| IBIS file stm32u535_545_lqfp64.ibs
[IBIS ver] 4.2
[File name] stm32u535_545_lqfp64.ibs
[File Rev] rev1.0
[Date]  11-09-2023
[Source] Data Created at STMicroelectronics
[Notes]  File originated from ELDO simulations.
[Disclaimer]  This information is for modeling purpose only and is
   not guaranteed. The information is subject to change without
   notice.
[Copyright] Copyright 2023 STMicroelectronics Inc.
|   Component stm32u535_545_lqfp64
[Component] stm32u535_545_lqfp64
[Manufacturer] STMicroelectronics
[Package]
| variable   typ   min   max
R_pkg  0  NA  NA
L_pkg  0  NA  NA
C_pkg  0  NA  NA
[Pin]   signal_name   model_name
1  VBAT  power
2  PC13  io8_100m_ft_v33
3  PC14-OSC32_IN  io8_100m_tamp_ft
4  PC15-OSC32_OUT  io8_100m_tamp_ft
5  PH0-OSC_IN  io8_100m_ft
6  PH1-OSC_OUT  io8_100m_ft
7  NRST  nc
8  PC0  io8_100m_hslv_i2c_ft
9  PC1  io8_166m_hslv_i2c_ft
10  PC2  io8_100m_hslv_ft
11  PC3  io8_100m_hslv_ft
12  VSSA  nc
13  VDDA  power
14  PA0  io8_100m_hslv_tamp_ft
15  PA1  io8_100m_hslv_tamp_ft
16  PA2  io8_100m_hslv_ft
17  PA3  io8_166m_hslv_ft
18  VSS  gnd
19  VDD  power
20  PA4  io8_100m_hslv_ft
21  PA5  io8_100m_ft
22  PA6  io8_100m_hslv_ft
23  PA7  io8_100m_hslv_i2c_ft
24  PC4  io8_100m_hslv_ft
25  PC5  io8_100m_tamp_ft
26  PB0  io8_100m_hslv_ft
27  PB1  io8_100m_hslv_ft
28  PB2  io8_100m_hslv_tamp_ft
29  PB10  io8_166m_hslv_i2c_ft
30  VCAP  nc
31  VSS  gnd
32  VDD  power
33  PB12  io8_166m_hslv_ft
34  PB13  io8_100m_i2c_ft
35  PB14  io8_100m_i2c_ft
36  PB15  io8_100m_ft
37  PC6  io8_100m_hslv_ft
38  PC7  io8_100m_hslv_ft
39  PC8  io8_100m_hslv_ft
40  PC9  io8_100m_hslv_ft
41  PA8  io8_166m_hslv_ft
42  PA9  io8_100m_ft
43  PA10  io8_100m_ft
44  PA11  io8_usb_ft
45  PA12  io8_usb_ft
46  PA13  io8_100m_ft
47  VSS  gnd
48  VDDUSB  power
49  PA14  io8_100m_ft
50  PA15  io8_100m_ft
51  PC10  io8_100m_hslv_ft
52  PC11  io8_100m_hslv_ft
53  PC12  io8_166m_hslv_ft
54  PD2  io8_100m_hslv_ft
55  PB3  io8_100m_i2c_ft
56  PB4  io8_100m_i2c_ft
57  PB5  io8_166m_hslv_ft
58  PB6  io8_100m_i2c_ft
59  PB7  io8_166m_hslv_i2c_ft
60  PH3-BOOT0  io8_100m_ft
61  PB8  io8_100m_hslv_i2c_ft
62  PB9  io8_100m_hslv_i2c_ft
63  VSS  gnd
64  VDD  power
[Package Model]   455-lqfp-10x10-64-ldo-230425
[Pin Mapping]   pulldown_ref   pullup_ref   | Comment
1  nc  vsw
2  gndio  vddiom  | Depending on IO usage
| 2  gndio  vsw  | Depending on IO usage
3  gndio  vddiom  | Depending on IO usage
| 3  gndio  vsw  | Depending on IO usage
4  gndio  vddiom  | Depending on IO usage
| 4  gndio  vsw  | Depending on IO usage
5  gndio  vddiom
6  gndio  vddiom
7  nc nc
8  gndio  vddiom
9  gndio  vddiom
10  gndio  vddiom
11  gndio  vddiom
12  nc  nc
13  nc  vddiom
14  gndio  vddiom
15  gndio  vddiom
16  gndio  vddiom
17  gndio  vddiom
18  gndio  nc
19  nc  vddiom
20  gndio  vddiom
21  gndio  vddiom
22  gndio  vddiom
23  gndio  vddiom
24  gndio  vddiom
25  gndio  vddiom
26  gndio  vddiom
27  gndio  vddiom
28  gndio  vddiom
29  gndio  vddiom
30  nc  nc
31  gndio  nc
32  nc  vddiom
33  gndio  vddiom
34  gndio  vddiom
35  gndio  vddiom
36  gndio  vddiom
37  gndio  vddiom
38  gndio  vddiom
39  gndio  vddiom
40  gndio  vddiom
41  gndio  vddiom
42  gndio  vddiom  | Depending on IO usage
| 42  gndio  vddusb  | Depending on IO usage
43  gndio  vddiom  | Depending on IO usage
| 43  gndio  vddusb  | Depending on IO usage
44  gndio  vddiom  | Depending on IO usage
| 44  gndio  vddusb  | Depending on IO usage
45  gndio  vddiom  | Depending on IO usage
| 45  gndio  vddusb  | Depending on IO usage
46  gndio  vddiom  | Depending on IO usage
| 46  gndio  vddusb  | Depending on IO usage
47  gndio  nc
48  nc  vddusb
49  gndio  vddiom
50  gndio  vddiom
51  gndio  vddiom
52  gndio  vddiom
53  gndio  vddiom
54  gndio  vddiom
55  gndio  vddiom
56  gndio  vddiom
57  gndio  vddiom
58  gndio  vddiom
59  gndio  vddiom
60  gndio  vddiom
61  gndio  vddiom
62  gndio  vddiom
63  gndio  nc
64  nc  vddiom
[Model Selector] io8_100m_ft
io8_100m_ft_hs_1v2  "IO8_FT 100MHz high speed @ 1.2V"
io8_100m_ft_fs_1v2  "IO8_FT 100MHz fast speed @ 1.2V"
io8_100m_ft_fs_pd_1v2  "IO8_FT 100MHz fast speed @ 1.2V pulldown"
io8_100m_ft_ms_1v2  "IO8_FT 100MHz med speed @ 1.2V"
io8_100m_ft_ms_pd_1v2  "IO8_FT 100MHz med speed @ 1.2V pulldown"
io8_100m_ft_ls_1v2  "IO8_FT 100MHz low speed @ 1.2V"
io8_100m_ft_ls_pd_1v2  "IO8_FT 100MHz low speed @ 1.2V pulldown"
io8_100m_ft_hs_1v8  "IO8_FT 100MHz high speed @ 1.8V"
io8_100m_ft_hs_pd_1v8  "IO8_FT 100MHz high speed @ 1.8V pulldown"
io8_100m_ft_fs_1v8  "IO8_FT 100MHz fast speed @ 1.8V"
io8_100m_ft_fs_pd_1v8  "IO8_FT 100MHz fast speed @ 1.8V pulldown"
io8_100m_ft_ms_1v8  "IO8_FT 100MHz med speed @ 1.8V"
io8_100m_ft_ms_pd_1v8  "IO8_FT 100MHz med speed @ 1.8V pulldown"
io8_100m_ft_ls_1v8  "IO8_FT 100MHz low speed @ 1.8V"
io8_100m_ft_ls_pd_1v8  "IO8_FT 100MHz low speed @ 1.8V pulldown"
io8_100m_ft_hs_3v3  "IO8_FT 100MHz high speed @ 3.3V"
io8_100m_ft_hs_pd_3v3  "IO8_FT 100MHz high speed @ 3.3V pulldown"
io8_100m_ft_fs_3v3  "IO8_FT 100MHz fast speed @ 3.3V"
io8_100m_ft_fs_pd_3v3  "IO8_FT 100MHz fast speed @ 3.3V pulldown"
io8_100m_ft_ms_3v3  "IO8_FT 100MHz med speed @ 3.3V"
io8_100m_ft_ms_pd_3v3  "IO8_FT 100MHz med speed @ 3.3V pulldown"
io8_100m_ft_ls_3v3  "IO8_FT 100MHz low speed @ 3.3V"
io8_100m_ft_ls_pd_3v3  "IO8_FT 100MHz low speed @ 3.3V pulldown"
[Model Selector] io8_100m_hslv_ft
io8_100m_ft_hs_1v2  "IO8_FT 100MHz high speed @ 1.2V"
io8_100m_ft_hs_pu_1v2  "IO8_FT 100MHz high speed @ 1.2V pullup"
io8_100m_ft_hs_pd_1v2  "IO8_FT 100MHz high speed @ 1.2V pulldown"
io8_100m_ft_fs_1v2  "IO8_FT 100MHz fast speed @ 1.2V"
io8_100m_ft_fs_pu_1v2  "IO8_FT 100MHz fast speed @ 1.2V pullup"
io8_100m_ft_fs_pd_1v2  "IO8_FT 100MHz fast speed @ 1.2V pulldown"
io8_100m_ft_ms_1v2  "IO8_FT 100MHz med speed @ 1.2V"
io8_100m_ft_ms_pu_1v2  "IO8_FT 100MHz med speed @ 1.2V pullup"
io8_100m_ft_ms_pd_1v2  "IO8_FT 100MHz med speed @ 1.2V pulldown"
io8_100m_ft_ls_1v2  "IO8_FT 100MHz low speed @ 1.2V"
io8_100m_ft_ls_pu_1v2  "IO8_FT 100MHz low speed @ 1.2V pullup"
io8_100m_ft_ls_pd_1v2  "IO8_FT 100MHz low speed @ 1.2V pulldown"
io8_100m_ft_hs_1v8  "IO8_FT 100MHz high speed @ 1.8V"
io8_100m_ft_hs_pu_1v8  "IO8_FT 100MHz high speed @ 1.8V pullup"
io8_100m_ft_hs_pd_1v8  "IO8_FT 100MHz high speed @ 1.8V pulldown"
io8_100m_ft_fs_1v8  "IO8_FT 100MHz fast speed @ 1.8V"
io8_100m_ft_fs_pu_1v8  "IO8_FT 100MHz fast speed @ 1.8V pullup"
io8_100m_ft_fs_pd_1v8  "IO8_FT 100MHz fast speed @ 1.8V pulldown"
io8_100m_ft_ms_1v8  "IO8_FT 100MHz med speed @ 1.8V"
io8_100m_ft_ms_pu_1v8  "IO8_FT 100MHz med speed @ 1.8V pullup"
io8_100m_ft_ms_pd_1v8  "IO8_FT 100MHz med speed @ 1.8V pulldown"
io8_100m_ft_ls_1v8  "IO8_FT 100MHz low speed @ 1.8V"
io8_100m_ft_ls_pu_1v8  "IO8_FT 100MHz low speed @ 1.8V pullup"
io8_100m_ft_ls_pd_1v8  "IO8_FT 100MHz low speed @ 1.8V pulldown"
io8_100m_ft_hs_3v3  "IO8_FT 100MHz high speed @ 3.3V"
io8_100m_ft_hs_pu_3v3  "IO8_FT 100MHz high speed @ 3.3V pullup"
io8_100m_ft_hs_pd_3v3  "IO8_FT 100MHz high speed @ 3.3V pulldown"
io8_100m_ft_fs_3v3  "IO8_FT 100MHz fast speed @ 3.3V"
io8_100m_ft_fs_pu_3v3  "IO8_FT 100MHz fast speed @ 3.3V pullup"
io8_100m_ft_fs_pd_3v3  "IO8_FT 100MHz fast speed @ 3.3V pulldown"
io8_100m_ft_ms_3v3  "IO8_FT 100MHz med speed @ 3.3V"
io8_100m_ft_ms_pu_3v3  "IO8_FT 100MHz med speed @ 3.3V pullup"
io8_100m_ft_ms_pd_3v3  "IO8_FT 100MHz med speed @ 3.3V pulldown"
io8_100m_ft_ls_3v3  "IO8_FT 100MHz low speed @ 3.3V"
io8_100m_ft_ls_pu_3v3  "IO8_FT 100MHz low speed @ 3.3V pullup"
io8_100m_ft_ls_pd_3v3  "IO8_FT 100MHz low speed @ 3.3V pulldown"
io8_100m_hslv_ft_hs_1v2  "IO8_FT 100MHz HSLV high speed @ 1.2V"
io8_100m_hslv_ft_hs_pu_1v2  "IO8_FT 100MHz HSLV high speed @ 1.2V pullup"
io8_100m_hslv_ft_hs_pd_1v2  "IO8_FT 100MHz HSLV high speed @ 1.2V pulldown"
io8_100m_hslv_ft_fs_1v2  "IO8_FT 100MHz HSLV fast speed @ 1.2V"
io8_100m_hslv_ft_fs_pu_1v2  "IO8_FT 100MHz HSLV fast speed @ 1.2V pullup"
io8_100m_hslv_ft_fs_pd_1v2  "IO8_FT 100MHz HSLV fast speed @ 1.2V pulldown"
io8_100m_hslv_ft_ms_1v2  "IO8_FT 100MHz HSLV med speed @ 1.2V"
io8_100m_hslv_ft_ms_pu_1v2  "IO8_FT 100MHz HSLV med speed @ 1.2V pullup"
io8_100m_hslv_ft_ms_pd_1v2  "IO8_FT 100MHz HSLV med speed @ 1.2V pulldown"
io8_100m_hslv_ft_ls_1v2  "IO8_FT 100MHz HSLV low speed @ 1.2V"
io8_100m_hslv_ft_ls_pu_1v2  "IO8_FT 100MHz HSLV low speed @ 1.2V pullup"
io8_100m_hslv_ft_ls_pd_1v2  "IO8_FT 100MHz HSLV low speed @ 1.2V pulldown"
io8_100m_hslv_ft_hs_1v8  "IO8_FT 100MHz HSLV high speed @ 1.8V"
io8_100m_hslv_ft_hs_pu_1v8  "IO8_FT 100MHz HSLV high speed @ 1.8V pullup"
io8_100m_hslv_ft_hs_pd_1v8  "IO8_FT 100MHz HSLV high speed @ 1.8V pulldown"
io8_100m_hslv_ft_fs_1v8  "IO8_FT 100MHz HSLV fast speed @ 1.8V"
io8_100m_hslv_ft_fs_pu_1v8  "IO8_FT 100MHz HSLV fast speed @ 1.8V pullup"
io8_100m_hslv_ft_fs_pd_1v8  "IO8_FT 100MHz HSLV fast speed @ 1.8V pulldown"
io8_100m_hslv_ft_ms_1v8  "IO8_FT 100MHz HSLV med speed @ 1.8V"
io8_100m_hslv_ft_ms_pu_1v8  "IO8_FT 100MHz HSLV med speed @ 1.8V pullup"
io8_100m_hslv_ft_ms_pd_1v8  "IO8_FT 100MHz HSLV med speed @ 1.8V pulldown"
io8_100m_hslv_ft_ls_1v8  "IO8_FT 100MHz HSLV low speed @ 1.8V"
io8_100m_hslv_ft_ls_pu_1v8  "IO8_FT 100MHz HSLV low speed @ 1.8V pullup"
io8_100m_hslv_ft_ls_pd_1v8  "IO8_FT 100MHz HSLV low speed @ 1.8V pulldown"
io8_100m_hslv_ft_hs_2v5  "IO8_FT 100MHz HSLV high speed @ 2.5V"
io8_100m_hslv_ft_hs_pu_2v5  "IO8_FT 100MHz HSLV high speed @ 2.5V pullup"
io8_100m_hslv_ft_hs_pd_2v5  "IO8_FT 100MHz HSLV high speed @ 2.5V pulldown"
io8_100m_hslv_ft_fs_2v5  "IO8_FT 100MHz HSLV fast speed @ 2.5V"
io8_100m_hslv_ft_fs_pu_2v5  "IO8_FT 100MHz HSLV fast speed @ 2.5V pullup"
io8_100m_hslv_ft_fs_pd_2v5  "IO8_FT 100MHz HSLV fast speed @ 2.5V pulldown"
io8_100m_hslv_ft_ms_2v5  "IO8_FT 100MHz HSLV med speed @ 2.5V"
io8_100m_hslv_ft_ms_pu_2v5  "IO8_FT 100MHz HSLV med speed @ 2.5V pullup"
io8_100m_hslv_ft_ms_pd_2v5  "IO8_FT 100MHz HSLV med speed @ 2.5V pulldown"
io8_100m_hslv_ft_ls_2v5  "IO8_FT 100MHz HSLV low speed @ 2.5V"
io8_100m_hslv_ft_ls_pu_2v5  "IO8_FT 100MHz HSLV low speed @ 2.5V pullup"
io8_100m_hslv_ft_ls_pd_2v5  "IO8_FT 100MHz HSLV low speed @ 2.5V pulldown"
[Model Selector] io8_100m_hslv_i2c_ft
io8_100m_ft_hs_1v2  "IO8_FT 100MHz high speed @ 1.2V"
io8_100m_ft_hs_pu_1v2  "IO8_FT 100MHz high speed @ 1.2V pullup"
io8_100m_ft_hs_pd_1v2  "IO8_FT 100MHz high speed @ 1.2V pulldown"
io8_100m_ft_fs_1v2  "IO8_FT 100MHz fast speed @ 1.2V"
io8_100m_ft_fs_pu_1v2  "IO8_FT 100MHz fast speed @ 1.2V pullup"
io8_100m_ft_fs_pd_1v2  "IO8_FT 100MHz fast speed @ 1.2V pulldown"
io8_100m_ft_ms_1v2  "IO8_FT 100MHz med speed @ 1.2V"
io8_100m_ft_ms_pu_1v2  "IO8_FT 100MHz med speed @ 1.2V pullup"
io8_100m_ft_ms_pd_1v2  "IO8_FT 100MHz med speed @ 1.2V pulldown"
io8_100m_ft_ls_1v2  "IO8_FT 100MHz low speed @ 1.2V"
io8_100m_ft_ls_pu_1v2  "IO8_FT 100MHz low speed @ 1.2V pullup"
io8_100m_ft_ls_pd_1v2  "IO8_FT 100MHz low speed @ 1.2V pulldown"
io8_100m_ft_hs_1v8  "IO8_FT 100MHz high speed @ 1.8V"
io8_100m_ft_hs_pu_1v8  "IO8_FT 100MHz high speed @ 1.8V pullup"
io8_100m_ft_hs_pd_1v8  "IO8_FT 100MHz high speed @ 1.8V pulldown"
io8_100m_ft_fs_1v8  "IO8_FT 100MHz fast speed @ 1.8V"
io8_100m_ft_fs_pu_1v8  "IO8_FT 100MHz fast speed @ 1.8V pullup"
io8_100m_ft_fs_pd_1v8  "IO8_FT 100MHz fast speed @ 1.8V pulldown"
io8_100m_ft_ms_1v8  "IO8_FT 100MHz med speed @ 1.8V"
io8_100m_ft_ms_pu_1v8  "IO8_FT 100MHz med speed @ 1.8V pullup"
io8_100m_ft_ms_pd_1v8  "IO8_FT 100MHz med speed @ 1.8V pulldown"
io8_100m_ft_ls_1v8  "IO8_FT 100MHz low speed @ 1.8V"
io8_100m_ft_ls_pu_1v8  "IO8_FT 100MHz low speed @ 1.8V pullup"
io8_100m_ft_ls_pd_1v8  "IO8_FT 100MHz low speed @ 1.8V pulldown"
io8_100m_ft_hs_3v3  "IO8_FT 100MHz high speed @ 3.3V"
io8_100m_ft_hs_pu_3v3  "IO8_FT 100MHz high speed @ 3.3V pullup"
io8_100m_ft_hs_pd_3v3  "IO8_FT 100MHz high speed @ 3.3V pulldown"
io8_100m_ft_fs_3v3  "IO8_FT 100MHz fast speed @ 3.3V"
io8_100m_ft_fs_pu_3v3  "IO8_FT 100MHz fast speed @ 3.3V pullup"
io8_100m_ft_fs_pd_3v3  "IO8_FT 100MHz fast speed @ 3.3V pulldown"
io8_100m_ft_ms_3v3  "IO8_FT 100MHz med speed @ 3.3V"
io8_100m_ft_ms_pu_3v3  "IO8_FT 100MHz med speed @ 3.3V pullup"
io8_100m_ft_ms_pd_3v3  "IO8_FT 100MHz med speed @ 3.3V pulldown"
io8_100m_ft_ls_3v3  "IO8_FT 100MHz low speed @ 3.3V"
io8_100m_ft_ls_pu_3v3  "IO8_FT 100MHz low speed @ 3.3V pullup"
io8_100m_ft_ls_pd_3v3  "IO8_FT 100MHz low speed @ 3.3V pulldown"
io8_100m_hslv_ft_hs_1v2  "IO8_FT 100MHz HSLV high speed @ 1.2V"
io8_100m_hslv_ft_hs_pu_1v2  "IO8_FT 100MHz HSLV high speed @ 1.2V pullup"
io8_100m_hslv_ft_hs_pd_1v2  "IO8_FT 100MHz HSLV high speed @ 1.2V pulldown"
io8_100m_hslv_ft_fs_1v2  "IO8_FT 100MHz HSLV fast speed @ 1.2V"
io8_100m_hslv_ft_fs_pu_1v2  "IO8_FT 100MHz HSLV fast speed @ 1.2V pullup"
io8_100m_hslv_ft_fs_pd_1v2  "IO8_FT 100MHz HSLV fast speed @ 1.2V pulldown"
io8_100m_hslv_ft_ms_1v2  "IO8_FT 100MHz HSLV med speed @ 1.2V"
io8_100m_hslv_ft_ms_pu_1v2  "IO8_FT 100MHz HSLV med speed @ 1.2V pullup"
io8_100m_hslv_ft_ms_pd_1v2  "IO8_FT 100MHz HSLV med speed @ 1.2V pulldown"
io8_100m_hslv_ft_ls_1v2  "IO8_FT 100MHz HSLV low speed @ 1.2V"
io8_100m_hslv_ft_ls_pu_1v2  "IO8_FT 100MHz HSLV low speed @ 1.2V pullup"
io8_100m_hslv_ft_ls_pd_1v2  "IO8_FT 100MHz HSLV low speed @ 1.2V pulldown"
io8_100m_hslv_ft_hs_1v8  "IO8_FT 100MHz HSLV high speed @ 1.8V"
io8_100m_hslv_ft_hs_pu_1v8  "IO8_FT 100MHz HSLV high speed @ 1.8V pullup"
io8_100m_hslv_ft_hs_pd_1v8  "IO8_FT 100MHz HSLV high speed @ 1.8V pulldown"
io8_100m_hslv_ft_fs_1v8  "IO8_FT 100MHz HSLV fast speed @ 1.8V"
io8_100m_hslv_ft_fs_pu_1v8  "IO8_FT 100MHz HSLV fast speed @ 1.8V pullup"
io8_100m_hslv_ft_fs_pd_1v8  "IO8_FT 100MHz HSLV fast speed @ 1.8V pulldown"
io8_100m_hslv_ft_ms_1v8  "IO8_FT 100MHz HSLV med speed @ 1.8V"
io8_100m_hslv_ft_ms_pu_1v8  "IO8_FT 100MHz HSLV med speed @ 1.8V pullup"
io8_100m_hslv_ft_ms_pd_1v8  "IO8_FT 100MHz HSLV med speed @ 1.8V pulldown"
io8_100m_hslv_ft_ls_1v8  "IO8_FT 100MHz HSLV low speed @ 1.8V"
io8_100m_hslv_ft_ls_pu_1v8  "IO8_FT 100MHz HSLV low speed @ 1.8V pullup"
io8_100m_hslv_ft_ls_pd_1v8  "IO8_FT 100MHz HSLV low speed @ 1.8V pulldown"
io8_100m_hslv_ft_hs_2v5  "IO8_FT 100MHz HSLV high speed @ 2.5V"
io8_100m_hslv_ft_hs_pu_2v5  "IO8_FT 100MHz HSLV high speed @ 2.5V pullup"
io8_100m_hslv_ft_hs_pd_2v5  "IO8_FT 100MHz HSLV high speed @ 2.5V pulldown"
io8_100m_hslv_ft_fs_2v5  "IO8_FT 100MHz HSLV fast speed @ 2.5V"
io8_100m_hslv_ft_fs_pu_2v5  "IO8_FT 100MHz HSLV fast speed @ 2.5V pullup"
io8_100m_hslv_ft_fs_pd_2v5  "IO8_FT 100MHz HSLV fast speed @ 2.5V pulldown"
io8_100m_hslv_ft_ms_2v5  "IO8_FT 100MHz HSLV med speed @ 2.5V"
io8_100m_hslv_ft_ms_pu_2v5  "IO8_FT 100MHz HSLV med speed @ 2.5V pullup"
io8_100m_hslv_ft_ms_pd_2v5  "IO8_FT 100MHz HSLV med speed @ 2.5V pulldown"
io8_100m_hslv_ft_ls_2v5  "IO8_FT 100MHz HSLV low speed @ 2.5V"
io8_100m_hslv_ft_ls_pu_2v5  "IO8_FT 100MHz HSLV low speed @ 2.5V pullup"
io8_100m_hslv_ft_ls_pd_2v5  "IO8_FT 100MHz HSLV low speed @ 2.5V pulldown"
[Model Selector] io8_100m_hslv_tamp_ft
io8_100m_ft_hs_1v2  "IO8_FT 100MHz high speed @ 1.2V"
io8_100m_ft_hs_pu_1v2  "IO8_FT 100MHz high speed @ 1.2V pullup"
io8_100m_ft_hs_pd_1v2  "IO8_FT 100MHz high speed @ 1.2V pulldown"
io8_100m_ft_fs_1v2  "IO8_FT 100MHz fast speed @ 1.2V"
io8_100m_ft_fs_pu_1v2  "IO8_FT 100MHz fast speed @ 1.2V pullup"
io8_100m_ft_fs_pd_1v2  "IO8_FT 100MHz fast speed @ 1.2V pulldown"
io8_100m_ft_ms_1v2  "IO8_FT 100MHz med speed @ 1.2V"
io8_100m_ft_ms_pu_1v2  "IO8_FT 100MHz med speed @ 1.2V pullup"
io8_100m_ft_ms_pd_1v2  "IO8_FT 100MHz med speed @ 1.2V pulldown"
io8_100m_ft_ls_1v2  "IO8_FT 100MHz low speed @ 1.2V"
io8_100m_ft_ls_pu_1v2  "IO8_FT 100MHz low speed @ 1.2V pullup"
io8_100m_ft_ls_pd_1v2  "IO8_FT 100MHz low speed @ 1.2V pulldown"
io8_100m_ft_hs_1v8  "IO8_FT 100MHz high speed @ 1.8V"
io8_100m_ft_hs_pu_1v8  "IO8_FT 100MHz high speed @ 1.8V pullup"
io8_100m_ft_hs_pd_1v8  "IO8_FT 100MHz high speed @ 1.8V pulldown"
io8_100m_ft_fs_1v8  "IO8_FT 100MHz fast speed @ 1.8V"
io8_100m_ft_fs_pu_1v8  "IO8_FT 100MHz fast speed @ 1.8V pullup"
io8_100m_ft_fs_pd_1v8  "IO8_FT 100MHz fast speed @ 1.8V pulldown"
io8_100m_ft_ms_1v8  "IO8_FT 100MHz med speed @ 1.8V"
io8_100m_ft_ms_pu_1v8  "IO8_FT 100MHz med speed @ 1.8V pullup"
io8_100m_ft_ms_pd_1v8  "IO8_FT 100MHz med speed @ 1.8V pulldown"
io8_100m_ft_ls_1v8  "IO8_FT 100MHz low speed @ 1.8V"
io8_100m_ft_ls_pu_1v8  "IO8_FT 100MHz low speed @ 1.8V pullup"
io8_100m_ft_ls_pd_1v8  "IO8_FT 100MHz low speed @ 1.8V pulldown"
io8_100m_ft_hs_3v3  "IO8_FT 100MHz high speed @ 3.3V"
io8_100m_ft_hs_pu_3v3  "IO8_FT 100MHz high speed @ 3.3V pullup"
io8_100m_ft_hs_pd_3v3  "IO8_FT 100MHz high speed @ 3.3V pulldown"
io8_100m_ft_fs_3v3  "IO8_FT 100MHz fast speed @ 3.3V"
io8_100m_ft_fs_pu_3v3  "IO8_FT 100MHz fast speed @ 3.3V pullup"
io8_100m_ft_fs_pd_3v3  "IO8_FT 100MHz fast speed @ 3.3V pulldown"
io8_100m_ft_ms_3v3  "IO8_FT 100MHz med speed @ 3.3V"
io8_100m_ft_ms_pu_3v3  "IO8_FT 100MHz med speed @ 3.3V pullup"
io8_100m_ft_ms_pd_3v3  "IO8_FT 100MHz med speed @ 3.3V pulldown"
io8_100m_ft_ls_3v3  "IO8_FT 100MHz low speed @ 3.3V"
io8_100m_ft_ls_pu_3v3  "IO8_FT 100MHz low speed @ 3.3V pullup"
io8_100m_ft_ls_pd_3v3  "IO8_FT 100MHz low speed @ 3.3V pulldown"
io8_100m_hslv_ft_hs_1v2  "IO8_FT 100MHz HSLV high speed @ 1.2V"
io8_100m_hslv_ft_hs_pu_1v2  "IO8_FT 100MHz HSLV high speed @ 1.2V pullup"
io8_100m_hslv_ft_hs_pd_1v2  "IO8_FT 100MHz HSLV high speed @ 1.2V pulldown"
io8_100m_hslv_ft_fs_1v2  "IO8_FT 100MHz HSLV fast speed @ 1.2V"
io8_100m_hslv_ft_fs_pu_1v2  "IO8_FT 100MHz HSLV fast speed @ 1.2V pullup"
io8_100m_hslv_ft_fs_pd_1v2  "IO8_FT 100MHz HSLV fast speed @ 1.2V pulldown"
io8_100m_hslv_ft_ms_1v2  "IO8_FT 100MHz HSLV med speed @ 1.2V"
io8_100m_hslv_ft_ms_pu_1v2  "IO8_FT 100MHz HSLV med speed @ 1.2V pullup"
io8_100m_hslv_ft_ms_pd_1v2  "IO8_FT 100MHz HSLV med speed @ 1.2V pulldown"
io8_100m_hslv_ft_ls_1v2  "IO8_FT 100MHz HSLV low speed @ 1.2V"
io8_100m_hslv_ft_ls_pu_1v2  "IO8_FT 100MHz HSLV low speed @ 1.2V pullup"
io8_100m_hslv_ft_ls_pd_1v2  "IO8_FT 100MHz HSLV low speed @ 1.2V pulldown"
io8_100m_hslv_ft_hs_1v8  "IO8_FT 100MHz HSLV high speed @ 1.8V"
io8_100m_hslv_ft_hs_pu_1v8  "IO8_FT 100MHz HSLV high speed @ 1.8V pullup"
io8_100m_hslv_ft_hs_pd_1v8  "IO8_FT 100MHz HSLV high speed @ 1.8V pulldown"
io8_100m_hslv_ft_fs_1v8  "IO8_FT 100MHz HSLV fast speed @ 1.8V"
io8_100m_hslv_ft_fs_pu_1v8  "IO8_FT 100MHz HSLV fast speed @ 1.8V pullup"
io8_100m_hslv_ft_fs_pd_1v8  "IO8_FT 100MHz HSLV fast speed @ 1.8V pulldown"
io8_100m_hslv_ft_ms_1v8  "IO8_FT 100MHz HSLV med speed @ 1.8V"
io8_100m_hslv_ft_ms_pu_1v8  "IO8_FT 100MHz HSLV med speed @ 1.8V pullup"
io8_100m_hslv_ft_ms_pd_1v8  "IO8_FT 100MHz HSLV med speed @ 1.8V pulldown"
io8_100m_hslv_ft_ls_1v8  "IO8_FT 100MHz HSLV low speed @ 1.8V"
io8_100m_hslv_ft_ls_pu_1v8  "IO8_FT 100MHz HSLV low speed @ 1.8V pullup"
io8_100m_hslv_ft_ls_pd_1v8  "IO8_FT 100MHz HSLV low speed @ 1.8V pulldown"
io8_100m_hslv_ft_hs_2v5  "IO8_FT 100MHz HSLV high speed @ 2.5V"
io8_100m_hslv_ft_hs_pu_2v5  "IO8_FT 100MHz HSLV high speed @ 2.5V pullup"
io8_100m_hslv_ft_hs_pd_2v5  "IO8_FT 100MHz HSLV high speed @ 2.5V pulldown"
io8_100m_hslv_ft_fs_2v5  "IO8_FT 100MHz HSLV fast speed @ 2.5V"
io8_100m_hslv_ft_fs_pu_2v5  "IO8_FT 100MHz HSLV fast speed @ 2.5V pullup"
io8_100m_hslv_ft_fs_pd_2v5  "IO8_FT 100MHz HSLV fast speed @ 2.5V pulldown"
io8_100m_hslv_ft_ms_2v5  "IO8_FT 100MHz HSLV med speed @ 2.5V"
io8_100m_hslv_ft_ms_pu_2v5  "IO8_FT 100MHz HSLV med speed @ 2.5V pullup"
io8_100m_hslv_ft_ms_pd_2v5  "IO8_FT 100MHz HSLV med speed @ 2.5V pulldown"
io8_100m_hslv_ft_ls_2v5  "IO8_FT 100MHz HSLV low speed @ 2.5V"
io8_100m_hslv_ft_ls_pu_2v5  "IO8_FT 100MHz HSLV low speed @ 2.5V pullup"
io8_100m_hslv_ft_ls_pd_2v5  "IO8_FT 100MHz HSLV low speed @ 2.5V pulldown"
io8_ft_v33_hs_1v2  "IO8_FT_V33 high speed @ 1.2V"
io8_ft_v33_hs_pu_1v2  "IO8_FT_V33 high speed @ 1.2V pullup"
io8_ft_v33_hs_pd_1v2  "IO8_FT_V33 high speed @ 1.2V pulldown"
io8_ft_v33_fs_1v2  "IO8_FT_V33 fast speed @ 1.2V"
io8_ft_v33_fs_pu_1v2  "IO8_FT_V33 fast speed @ 1.2V pullup"
io8_ft_v33_fs_pd_1v2  "IO8_FT_V33 fast speed @ 1.2V pulldown"
io8_ft_v33_ms_1v2  "IO8_FT_V33 med speed @ 1.2V"
io8_ft_v33_ms_pu_1v2  "IO8_FT_V33 med speed @ 1.2V pullup"
io8_ft_v33_ms_pd_1v2  "IO8_FT_V33 med speed @ 1.2V pulldown"
io8_ft_v33_ls_1v2  "IO8_FT_V33 low speed @ 1.2V"
io8_ft_v33_ls_pu_1v2  "IO8_FT_V33 low speed @ 1.2V pullup"
io8_ft_v33_ls_pd_1v2  "IO8_FT_V33 low speed @ 1.2V pulldown"
io8_ft_v33_hs_1v8  "IO8_FT_V33 high speed @ 1.8V"
io8_ft_v33_hs_pu_1v8  "IO8_FT_V33 high speed @ 1.8V pullup"
io8_ft_v33_hs_pd_1v8  "IO8_FT_V33 high speed @ 1.8V pulldown"
io8_ft_v33_fs_1v8  "IO8_FT_V33 fast speed @ 1.8V"
io8_ft_v33_fs_pu_1v8  "IO8_FT_V33 fast speed @ 1.8V pullup"
io8_ft_v33_fs_pd_1v8  "IO8_FT_V33 fast speed @ 1.8V pulldown"
io8_ft_v33_ms_1v8  "IO8_FT_V33 med speed @ 1.8V"
io8_ft_v33_ms_pu_1v8  "IO8_FT_V33 med speed @ 1.8V pullup"
io8_ft_v33_ms_pd_1v8  "IO8_FT_V33 med speed @ 1.8V pulldown"
io8_ft_v33_ls_1v8  "IO8_FT_V33 low speed @ 1.8V"
io8_ft_v33_ls_pu_1v8  "IO8_FT_V33 low speed @ 1.8V pullup"
io8_ft_v33_ls_pd_1v8  "IO8_FT_V33 low speed @ 1.8V pulldown"
io8_ft_v33_hs_3v3  "IO8_FT_V33 high speed @ 3.3V"
io8_ft_v33_hs_pu_3v3  "IO8_FT_V33 high speed @ 3.3V pullup"
io8_ft_v33_hs_pd_3v3  "IO8_FT_V33 high speed @ 3.3V pulldown"
io8_ft_v33_fs_3v3  "IO8_FT_V33 fast speed @ 3.3V"
io8_ft_v33_fs_pu_3v3  "IO8_FT_V33 fast speed @ 3.3V pullup"
io8_ft_v33_fs_pd_3v3  "IO8_FT_V33 fast speed @ 3.3V pulldown"
io8_ft_v33_ms_3v3  "IO8_FT_V33 med speed @ 3.3V"
io8_ft_v33_ms_pu_3v3  "IO8_FT_V33 med speed @ 3.3V pullup"
io8_ft_v33_ms_pd_3v3  "IO8_FT_V33 med speed @ 3.3V pulldown"
io8_ft_v33_ls_3v3  "IO8_FT_V33 low speed @ 3.3V"
io8_ft_v33_ls_pu_3v3  "IO8_FT_V33 low speed @ 3.3V pullup"
io8_ft_v33_ls_pd_3v3  "IO8_FT_V33 low speed @ 3.3V pulldown"
[Model Selector] io8_100m_i2c_ft
io8_100m_ft_hs_1v2  "IO8_FT 100MHz high speed @ 1.2V"
io8_100m_ft_hs_pu_1v2  "IO8_FT 100MHz high speed @ 1.2V pullup"
io8_100m_ft_hs_pd_1v2  "IO8_FT 100MHz high speed @ 1.2V pulldown"
io8_100m_ft_fs_1v2  "IO8_FT 100MHz fast speed @ 1.2V"
io8_100m_ft_fs_pu_1v2  "IO8_FT 100MHz fast speed @ 1.2V pullup"
io8_100m_ft_fs_pd_1v2  "IO8_FT 100MHz fast speed @ 1.2V pulldown"
io8_100m_ft_ms_1v2  "IO8_FT 100MHz med speed @ 1.2V"
io8_100m_ft_ms_pu_1v2  "IO8_FT 100MHz med speed @ 1.2V pullup"
io8_100m_ft_ms_pd_1v2  "IO8_FT 100MHz med speed @ 1.2V pulldown"
io8_100m_ft_ls_1v2  "IO8_FT 100MHz low speed @ 1.2V"
io8_100m_ft_ls_pu_1v2  "IO8_FT 100MHz low speed @ 1.2V pullup"
io8_100m_ft_ls_pd_1v2  "IO8_FT 100MHz low speed @ 1.2V pulldown"
io8_100m_ft_hs_1v8  "IO8_FT 100MHz high speed @ 1.8V"
io8_100m_ft_hs_pu_1v8  "IO8_FT 100MHz high speed @ 1.8V pullup"
io8_100m_ft_hs_pd_1v8  "IO8_FT 100MHz high speed @ 1.8V pulldown"
io8_100m_ft_fs_1v8  "IO8_FT 100MHz fast speed @ 1.8V"
io8_100m_ft_fs_pu_1v8  "IO8_FT 100MHz fast speed @ 1.8V pullup"
io8_100m_ft_fs_pd_1v8  "IO8_FT 100MHz fast speed @ 1.8V pulldown"
io8_100m_ft_ms_1v8  "IO8_FT 100MHz med speed @ 1.8V"
io8_100m_ft_ms_pu_1v8  "IO8_FT 100MHz med speed @ 1.8V pullup"
io8_100m_ft_ms_pd_1v8  "IO8_FT 100MHz med speed @ 1.8V pulldown"
io8_100m_ft_ls_1v8  "IO8_FT 100MHz low speed @ 1.8V"
io8_100m_ft_ls_pu_1v8  "IO8_FT 100MHz low speed @ 1.8V pullup"
io8_100m_ft_ls_pd_1v8  "IO8_FT 100MHz low speed @ 1.8V pulldown"
io8_100m_ft_hs_3v3  "IO8_FT 100MHz high speed @ 3.3V"
io8_100m_ft_hs_pu_3v3  "IO8_FT 100MHz high speed @ 3.3V pullup"
io8_100m_ft_hs_pd_3v3  "IO8_FT 100MHz high speed @ 3.3V pulldown"
io8_100m_ft_fs_3v3  "IO8_FT 100MHz fast speed @ 3.3V"
io8_100m_ft_fs_pu_3v3  "IO8_FT 100MHz fast speed @ 3.3V pullup"
io8_100m_ft_fs_pd_3v3  "IO8_FT 100MHz fast speed @ 3.3V pulldown"
io8_100m_ft_ms_3v3  "IO8_FT 100MHz med speed @ 3.3V"
io8_100m_ft_ms_pu_3v3  "IO8_FT 100MHz med speed @ 3.3V pullup"
io8_100m_ft_ms_pd_3v3  "IO8_FT 100MHz med speed @ 3.3V pulldown"
io8_100m_ft_ls_3v3  "IO8_FT 100MHz low speed @ 3.3V"
io8_100m_ft_ls_pu_3v3  "IO8_FT 100MHz low speed @ 3.3V pullup"
io8_100m_ft_ls_pd_3v3  "IO8_FT 100MHz low speed @ 3.3V pulldown"
io8_100m_i2c_ft_1v2  "IO8_FT 100MHz I2C @ 1.2V"
io8_100m_i2c_ft_pu_1v2  "IO8_FT 100MHz I2C @ 1.2V pullup"
io8_100m_i2c_ft_pd_1v2  "IO8_FT 100MHz I2C @ 1.2V pulldown"
io8_100m_i2c_ft_1v8  "IO8_FT 100MHz I2C @ 1.8V"
io8_100m_i2c_ft_pu_1v8  "IO8_FT 100MHz I2C @ 1.8V pullup"
io8_100m_i2c_ft_pd_1v8  "IO8_FT 100MHz I2C @ 1,8V pulldown"
io8_100m_i2c_ft_3v3  "IO8_FT 100MHz I2C @ 3.3V"
io8_100m_i2c_ft_pu_3v3  "IO8_FT 100MHz I2C HSLV @ 3.3V pullup"
io8_100m_i2c_ft_pd_3v3  "IO8_FT 100MHz I2C @ 3.3V pulldown"
[Model Selector] io8_100m_tamp_ft
io8_100m_ft_hs_1v2  "IO8_FT 100MHz high speed @ 1.2V"
io8_100m_ft_hs_pu_1v2  "IO8_FT 100MHz high speed @ 1.2V pullup"
io8_100m_ft_hs_pd_1v2  "IO8_FT 100MHz high speed @ 1.2V pulldown"
io8_100m_ft_fs_1v2  "IO8_FT 100MHz fast speed @ 1.2V"
io8_100m_ft_fs_pu_1v2  "IO8_FT 100MHz fast speed @ 1.2V pullup"
io8_100m_ft_fs_pd_1v2  "IO8_FT 100MHz fast speed @ 1.2V pulldown"
io8_100m_ft_ms_1v2  "IO8_FT 100MHz med speed @ 1.2V"
io8_100m_ft_ms_pu_1v2  "IO8_FT 100MHz med speed @ 1.2V pullup"
io8_100m_ft_ms_pd_1v2  "IO8_FT 100MHz med speed @ 1.2V pulldown"
io8_100m_ft_ls_1v2  "IO8_FT 100MHz low speed @ 1.2V"
io8_100m_ft_ls_pu_1v2  "IO8_FT 100MHz low speed @ 1.2V pullup"
io8_100m_ft_ls_pd_1v2  "IO8_FT 100MHz low speed @ 1.2V pulldown"
io8_100m_ft_hs_1v8  "IO8_FT 100MHz high speed @ 1.8V"
io8_100m_ft_hs_pu_1v8  "IO8_FT 100MHz high speed @ 1.8V pullup"
io8_100m_ft_hs_pd_1v8  "IO8_FT 100MHz high speed @ 1.8V pulldown"
io8_100m_ft_fs_1v8  "IO8_FT 100MHz fast speed @ 1.8V"
io8_100m_ft_fs_pu_1v8  "IO8_FT 100MHz fast speed @ 1.8V pullup"
io8_100m_ft_fs_pd_1v8  "IO8_FT 100MHz fast speed @ 1.8V pulldown"
io8_100m_ft_ms_1v8  "IO8_FT 100MHz med speed @ 1.8V"
io8_100m_ft_ms_pu_1v8  "IO8_FT 100MHz med speed @ 1.8V pullup"
io8_100m_ft_ms_pd_1v8  "IO8_FT 100MHz med speed @ 1.8V pulldown"
io8_100m_ft_ls_1v8  "IO8_FT 100MHz low speed @ 1.8V"
io8_100m_ft_ls_pu_1v8  "IO8_FT 100MHz low speed @ 1.8V pullup"
io8_100m_ft_ls_pd_1v8  "IO8_FT 100MHz low speed @ 1.8V pulldown"
io8_100m_ft_hs_3v3  "IO8_FT 100MHz high speed @ 3.3V"
io8_100m_ft_hs_pu_3v3  "IO8_FT 100MHz high speed @ 3.3V pullup"
io8_100m_ft_hs_pd_3v3  "IO8_FT 100MHz high speed @ 3.3V pulldown"
io8_100m_ft_fs_3v3  "IO8_FT 100MHz fast speed @ 3.3V"
io8_100m_ft_fs_pu_3v3  "IO8_FT 100MHz fast speed @ 3.3V pullup"
io8_100m_ft_fs_pd_3v3  "IO8_FT 100MHz fast speed @ 3.3V pulldown"
io8_100m_ft_ms_3v3  "IO8_FT 100MHz med speed @ 3.3V"
io8_100m_ft_ms_pu_3v3  "IO8_FT 100MHz med speed @ 3.3V pullup"
io8_100m_ft_ms_pd_3v3  "IO8_FT 100MHz med speed @ 3.3V pulldown"
io8_100m_ft_ls_3v3  "IO8_FT 100MHz low speed @ 3.3V"
io8_100m_ft_ls_pu_3v3  "IO8_FT 100MHz low speed @ 3.3V pullup"
io8_100m_ft_ls_pd_3v3  "IO8_FT 100MHz low speed @ 3.3V pulldown"
io8_ft_v33_hs_1v2  "IO8_FT_V33 high speed @ 1.2V"
io8_ft_v33_hs_pu_1v2  "IO8_FT_V33 high speed @ 1.2V pullup"
io8_ft_v33_hs_pd_1v2  "IO8_FT_V33 high speed @ 1.2V pulldown"
io8_ft_v33_fs_1v2  "IO8_FT_V33 fast speed @ 1.2V"
io8_ft_v33_fs_pu_1v2  "IO8_FT_V33 fast speed @ 1.2V pullup"
io8_ft_v33_fs_pd_1v2  "IO8_FT_V33 fast speed @ 1.2V pulldown"
io8_ft_v33_ms_1v2  "IO8_FT_V33 med speed @ 1.2V"
io8_ft_v33_ms_pu_1v2  "IO8_FT_V33 med speed @ 1.2V pullup"
io8_ft_v33_ms_pd_1v2  "IO8_FT_V33 med speed @ 1.2V pulldown"
io8_ft_v33_ls_1v2  "IO8_FT_V33 low speed @ 1.2V"
io8_ft_v33_ls_pu_1v2  "IO8_FT_V33 low speed @ 1.2V pullup"
io8_ft_v33_ls_pd_1v2  "IO8_FT_V33 low speed @ 1.2V pulldown"
io8_ft_v33_hs_1v8  "IO8_FT_V33 high speed @ 1.8V"
io8_ft_v33_hs_pu_1v8  "IO8_FT_V33 high speed @ 1.8V pullup"
io8_ft_v33_hs_pd_1v8  "IO8_FT_V33 high speed @ 1.8V pulldown"
io8_ft_v33_fs_1v8  "IO8_FT_V33 fast speed @ 1.8V"
io8_ft_v33_fs_pu_1v8  "IO8_FT_V33 fast speed @ 1.8V pullup"
io8_ft_v33_fs_pd_1v8  "IO8_FT_V33 fast speed @ 1.8V pulldown"
io8_ft_v33_ms_1v8  "IO8_FT_V33 med speed @ 1.8V"
io8_ft_v33_ms_pu_1v8  "IO8_FT_V33 med speed @ 1.8V pullup"
io8_ft_v33_ms_pd_1v8  "IO8_FT_V33 med speed @ 1.8V pulldown"
io8_ft_v33_ls_1v8  "IO8_FT_V33 low speed @ 1.8V"
io8_ft_v33_ls_pu_1v8  "IO8_FT_V33 low speed @ 1.8V pullup"
io8_ft_v33_ls_pd_1v8  "IO8_FT_V33 low speed @ 1.8V pulldown"
io8_ft_v33_hs_3v3  "IO8_FT_V33 high speed @ 3.3V"
io8_ft_v33_hs_pu_3v3  "IO8_FT_V33 high speed @ 3.3V pullup"
io8_ft_v33_hs_pd_3v3  "IO8_FT_V33 high speed @ 3.3V pulldown"
io8_ft_v33_fs_3v3  "IO8_FT_V33 fast speed @ 3.3V"
io8_ft_v33_fs_pu_3v3  "IO8_FT_V33 fast speed @ 3.3V pullup"
io8_ft_v33_fs_pd_3v3  "IO8_FT_V33 fast speed @ 3.3V pulldown"
io8_ft_v33_ms_3v3  "IO8_FT_V33 med speed @ 3.3V"
io8_ft_v33_ms_pu_3v3  "IO8_FT_V33 med speed @ 3.3V pullup"
io8_ft_v33_ms_pd_3v3  "IO8_FT_V33 med speed @ 3.3V pulldown"
io8_ft_v33_ls_3v3  "IO8_FT_V33 low speed @ 3.3V"
io8_ft_v33_ls_pu_3v3  "IO8_FT_V33 low speed @ 3.3V pullup"
io8_ft_v33_ls_pd_3v3  "IO8_FT_V33 low speed @ 3.3V pulldown"
[Model Selector] io8_usb_ft
io8_100m_ft_hs_1v2  "IO8_FT 100MHz high speed @ 1.2V"
io8_100m_ft_hs_pu_1v2  "IO8_FT 100MHz high speed @ 1.2V pullup"
io8_100m_ft_hs_pd_1v2  "IO8_FT 100MHz high speed @ 1.2V pulldown"
io8_100m_ft_fs_1v2  "IO8_FT 100MHz fast speed @ 1.2V"
io8_100m_ft_fs_pu_1v2  "IO8_FT 100MHz fast speed @ 1.2V pullup"
io8_100m_ft_fs_pd_1v2  "IO8_FT 100MHz fast speed @ 1.2V pulldown"
io8_100m_ft_ms_1v2  "IO8_FT 100MHz med speed @ 1.2V"
io8_100m_ft_ms_pu_1v2  "IO8_FT 100MHz med speed @ 1.2V pullup"
io8_100m_ft_ms_pd_1v2  "IO8_FT 100MHz med speed @ 1.2V pulldown"
io8_100m_ft_ls_1v2  "IO8_FT 100MHz low speed @ 1.2V"
io8_100m_ft_ls_pu_1v2  "IO8_FT 100MHz low speed @ 1.2V pullup"
io8_100m_ft_ls_pd_1v2  "IO8_FT 100MHz low speed @ 1.2V pulldown"
io8_100m_ft_hs_1v8  "IO8_FT 100MHz high speed @ 1.8V"
io8_100m_ft_hs_pu_1v8  "IO8_FT 100MHz high speed @ 1.8V pullup"
io8_100m_ft_hs_pd_1v8  "IO8_FT 100MHz high speed @ 1.8V pulldown"
io8_100m_ft_fs_1v8  "IO8_FT 100MHz fast speed @ 1.8V"
io8_100m_ft_fs_pu_1v8  "IO8_FT 100MHz fast speed @ 1.8V pullup"
io8_100m_ft_fs_pd_1v8  "IO8_FT 100MHz fast speed @ 1.8V pulldown"
io8_100m_ft_ms_1v8  "IO8_FT 100MHz med speed @ 1.8V"
io8_100m_ft_ms_pu_1v8  "IO8_FT 100MHz med speed @ 1.8V pullup"
io8_100m_ft_ms_pd_1v8  "IO8_FT 100MHz med speed @ 1.8V pulldown"
io8_100m_ft_ls_1v8  "IO8_FT 100MHz low speed @ 1.8V"
io8_100m_ft_ls_pu_1v8  "IO8_FT 100MHz low speed @ 1.8V pullup"
io8_100m_ft_ls_pd_1v8  "IO8_FT 100MHz low speed @ 1.8V pulldown"
io8_100m_ft_hs_3v3  "IO8_FT 100MHz high speed @ 3.3V"
io8_100m_ft_hs_pu_3v3  "IO8_FT 100MHz high speed @ 3.3V pullup"
io8_100m_ft_hs_pd_3v3  "IO8_FT 100MHz high speed @ 3.3V pulldown"
io8_100m_ft_fs_3v3  "IO8_FT 100MHz fast speed @ 3.3V"
io8_100m_ft_fs_pu_3v3  "IO8_FT 100MHz fast speed @ 3.3V pullup"
io8_100m_ft_fs_pd_3v3  "IO8_FT 100MHz fast speed @ 3.3V pulldown"
io8_100m_ft_ms_3v3  "IO8_FT 100MHz med speed @ 3.3V"
io8_100m_ft_ms_pu_3v3  "IO8_FT 100MHz med speed @ 3.3V pullup"
io8_100m_ft_ms_pd_3v3  "IO8_FT 100MHz med speed @ 3.3V pulldown"
io8_100m_ft_ls_3v3  "IO8_FT 100MHz low speed @ 3.3V"
io8_100m_ft_ls_pu_3v3  "IO8_FT 100MHz low speed @ 3.3V pullup"
io8_100m_ft_ls_pd_3v3  "IO8_FT 100MHz low speed @ 3.3V pulldown"
io8_usb_fs_3v3  "IOUSB fast speed @ 3.3V"
io8_usb_fs_pu1_3v3  "IO8USB fast speed @ 3.3V pullup1"
io8_usb_fs_pd1_3v3  "IOUSB fast speed @ 3.3V pulldown1"
io8_usb_ls_3v3  "IOUSB low speed @ 3.3V"
io8_usb_ls_pu1_3v3  "IOUSB low speed @ 3.3V pullup1"
io8_usb_ls_pd1_3v3  "IOUSB low speed @ 3.3V pulldown1"
io8_usb_fs_pu2_3v3  "IOUSB fast speed @ 3.3V pullup2"
io8_usb_fs_pd2_3v3  "IOUSB fast speed @ 3.3V pulldown2"
io8_usb_ls_pu2_3v3  "IOUSB low speed @ 3.3V pullup2"
io8_usb_ls_pd2_3v3  "IOUSB low speed @ 3.3V pulldown2"
[Model Selector] io8_166m_hslv_ft
io8_166m_ft_hs_1v2  "IO8_FT 166MHz high speed @ 1.2V"
io8_166m_ft_hs_pu_1v2  "IO8_FT 166MHz high speed @ 1.2V pullup"
io8_166m_ft_hs_pd_1v2  "IO8_FT 166MHz high speed @ 1.2V pulldown"
io8_166m_ft_fs_1v2  "IO8_FT 166MHz fast speed @ 1.2V"
io8_166m_ft_fs_pu_1v2  "IO8_FT 166MHz fast speed @ 1.2V pullup"
io8_166m_ft_fs_pd_1v2  "IO8_FT 166MHz fast speed @ 1.2V pulldown"
io8_166m_ft_ms_1v2  "IO8_FT 166MHz med speed @ 1.2V"
io8_166m_ft_ms_pu_1v2  "IO8_FT 166MHz med speed @ 1.2V pullup"
io8_166m_ft_ms_pd_1v2  "IO8_FT 166MHz med speed @ 1.2V pulldown"
io8_166m_ft_ls_1v2  "IO8_FT 166MHz low speed @ 1.2V"
io8_166m_ft_ls_pu_1v2  "IO8_FT 166MHz low speed @ 1.2V pullup"
io8_166m_ft_ls_pd_1v2  "IO8_FT 166MHz low speed @ 1.2V pulldown"
io8_166m_ft_hs_1v8  "IO8_FT 166MHz high speed @ 1.8V"
io8_166m_ft_hs_pu_1v8  "IO8_FT 166MHz high speed @ 1.8V pullup"
io8_166m_ft_hs_pd_1v8  "IO8_FT 166MHz high speed @ 1.8V pulldown"
io8_166m_ft_fs_1v8  "IO8_FT 166MHz fast speed @ 1.8V"
io8_166m_ft_fs_pu_1v8  "IO8_FT 166MHz fast speed @ 1.8V pullup"
io8_166m_ft_fs_pd_1v8  "IO8_FT 166MHz fast speed @ 1.8V pulldown"
io8_166m_ft_ms_1v8  "IO8_FT 166MHz med speed @ 1.8V"
io8_166m_ft_ms_pu_1v8  "IO8_FT 166MHz med speed @ 1.8V pullup"
io8_166m_ft_ms_pd_1v8  "IO8_FT 166MHz med speed @ 1.8V pulldown"
io8_166m_ft_ls_1v8  "IO8_FT 166MHz low speed @ 1.8V"
io8_166m_ft_ls_pu_1v8  "IO8_FT 166MHz low speed @ 1.8V pullup"
io8_166m_ft_ls_pd_1v8  "IO8_FT 166MHz low speed @ 1.8V pulldown"
io8_166m_ft_hs_3v3  "IO8_FT 166MHz high speed @ 3.3V"
io8_166m_ft_hs_pu_3v3  "IO8_FT 166MHz high speed @ 3.3V pullup"
io8_166m_ft_hs_pd_3v3  "IO8_FT 166MHz high speed @ 3.3V pulldown"
io8_166m_ft_fs_3v3  "IO8_FT 166MHz fast speed @ 3.3V"
io8_166m_ft_fs_pu_3v3  "IO8_FT 166MHz fast speed @ 3.3V pullup"
io8_166m_ft_fs_pd_3v3  "IO8_FT 166MHz fast speed @ 3.3V pulldown"
io8_166m_ft_ms_3v3  "IO8_FT 166MHz med speed @ 3.3V"
io8_166m_ft_ms_pu_3v3  "IO8_FT 166MHz med speed @ 3.3V pullup"
io8_166m_ft_ms_pd_3v3  "IO8_FT 166MHz med speed @ 3.3V pulldown"
io8_166m_ft_ls_3v3  "IO8_FT 166MHz low speed @ 3.3V"
io8_166m_ft_ls_pu_3v3  "IO8_FT 166MHz low speed @ 3.3V pullup"
io8_166m_ft_ls_pd_3v3  "IO8_FT 166MHz low speed @ 3.3V pulldown"
io8_166m_hslv_ft_hs_1v2  "IO8_FT 166MHz HSLV high speed @ 1.2V"
io8_166m_hslv_ft_hs_pu_1v2  "IO8_FT 166MHz HSLV high speed @ 1.2V pullup"
io8_166m_hslv_ft_hs_pd_1v2  "IO8_FT 166MHz HSLV high speed @ 1.2V pulldown"
io8_166m_hslv_ft_fs_1v2  "IO8_FT 166MHz HSLV fast speed @ 1.2V"
io8_166m_hslv_ft_fs_pu_1v2  "IO8_FT 166MHz HSLV fast speed @ 1.2V pullup"
io8_166m_hslv_ft_fs_pd_1v2  "IO8_FT 166MHz HSLV fast speed @ 1.2V pulldown"
io8_166m_hslv_ft_ms_1v2  "IO8_FT 166MHz HSLV med speed @ 1.2V"
io8_166m_hslv_ft_ms_pu_1v2  "IO8_FT 166MHz HSLV med speed @ 1.2V pullup"
io8_166m_hslv_ft_ms_pd_1v2  "IO8_FT 166MHz HSLV med speed @ 1.2V pulldown"
io8_166m_hslv_ft_ls_1v2  "IO8_FT 166MHz HSLV low speed @ 1.2V"
io8_166m_hslv_ft_ls_pu_1v2  "IO8_FT 166MHz HSLV low speed @ 1.2V pullup"
io8_166m_hslv_ft_ls_pd_1v2  "IO8_FT 166MHz HSLV low speed @ 1.2V pulldown"
io8_166m_hslv_ft_hs_1v8  "IO8_FT 166MHz HSLV high speed @ 1.8V"
io8_166m_hslv_ft_hs_pu_1v8  "IO8_FT 166MHz HSLV high speed @ 1.8V pullup"
io8_166m_hslv_ft_hs_pd_1v8  "IO8_FT 166MHz HSLV high speed @ 1.8V pulldown"
io8_166m_hslv_ft_fs_1v8  "IO8_FT 166MHz HSLV fast speed @ 1.8V"
io8_166m_hslv_ft_fs_pu_1v8  "IO8_FT 166MHz HSLV fast speed @ 1.8V pullup"
io8_166m_hslv_ft_fs_pd_1v8  "IO8_FT 166MHz HSLV fast speed @ 1.8V pulldown"
io8_166m_hslv_ft_ms_1v8  "IO8_FT 166MHz HSLV med speed @ 1.8V"
io8_166m_hslv_ft_ms_pu_1v8  "IO8_FT 166MHz HSLV med speed @ 1.8V pullup"
io8_166m_hslv_ft_ms_pd_1v8  "IO8_FT 166MHz HSLV med speed @ 1.8V pulldown"
io8_166m_hslv_ft_ls_1v8  "IO8_FT 166MHz HSLV low speed @ 1.8V"
io8_166m_hslv_ft_ls_pu_1v8  "IO8_FT 166MHz HSLV low speed @ 1.8V pullup"
io8_166m_hslv_ft_ls_pd_1v8  "IO8_FT 166MHz HSLV low speed @ 1.8V pulldown"
io8_166m_hslv_ft_hs_2v5  "IO8_FT 166MHz HSLV high speed @ 2.5V"
io8_166m_hslv_ft_hs_pu_2v5  "IO8_FT 166MHz HSLV high speed @ 2.5V pullup"
io8_166m_hslv_ft_hs_pd_2v5  "IO8_FT 166MHz HSLV high speed @ 2.5V pulldown"
io8_166m_hslv_ft_fs_2v5  "IO8_FT 166MHz HSLV fast speed @ 2.5V"
io8_166m_hslv_ft_fs_pu_2v5  "IO8_FT 166MHz HSLV fast speed @ 2.5V pullup"
io8_166m_hslv_ft_fs_pd_2v5  "IO8_FT 166MHz HSLV fast speed @ 2.5V pulldown"
io8_166m_hslv_ft_ms_2v5  "IO8_FT 166MHz HSLV med speed @ 2.5V"
io8_166m_hslv_ft_ms_pu_2v5  "IO8_FT 166MHz HSLV med speed @ 2.5V pullup"
io8_166m_hslv_ft_ms_pd_2v5  "IO8_FT 166MHz HSLV med speed @ 2.5V pulldown"
io8_166m_hslv_ft_ls_2v5  "IO8_FT 166MHz HSLV low speed @ 2.5V"
io8_166m_hslv_ft_ls_pu_2v5  "IO8_FT 166MHz HSLV low speed @ 2.5V pullup"
io8_166m_hslv_ft_ls_pd_2v5  "IO8_FT 166MHz HSLV low speed @ 2.5V pulldown"
[Model Selector] io8_166m_hslv_i2c_ft
io8_166m_ft_hs_1v2  "IO8_FT 166MHz high speed @ 1.2V"
io8_166m_ft_hs_pu_1v2  "IO8_FT 166MHz high speed @ 1.2V pullup"
io8_166m_ft_hs_pd_1v2  "IO8_FT 166MHz high speed @ 1.2V pulldown"
io8_166m_ft_fs_1v2  "IO8_FT 166MHz fast speed @ 1.2V"
io8_166m_ft_fs_pu_1v2  "IO8_FT 166MHz fast speed @ 1.2V pullup"
io8_166m_ft_fs_pd_1v2  "IO8_FT 166MHz fast speed @ 1.2V pulldown"
io8_166m_ft_ms_1v2  "IO8_FT 166MHz med speed @ 1.2V"
io8_166m_ft_ms_pu_1v2  "IO8_FT 166MHz med speed @ 1.2V pullup"
io8_166m_ft_ms_pd_1v2  "IO8_FT 166MHz med speed @ 1.2V pulldown"
io8_166m_ft_ls_1v2  "IO8_FT 166MHz low speed @ 1.2V"
io8_166m_ft_ls_pu_1v2  "IO8_FT 166MHz low speed @ 1.2V pullup"
io8_166m_ft_ls_pd_1v2  "IO8_FT 166MHz low speed @ 1.2V pulldown"
io8_166m_ft_hs_1v8  "IO8_FT 166MHz high speed @ 1.8V"
io8_166m_ft_hs_pu_1v8  "IO8_FT 166MHz high speed @ 1.8V pullup"
io8_166m_ft_hs_pd_1v8  "IO8_FT 166MHz high speed @ 1.8V pulldown"
io8_166m_ft_fs_1v8  "IO8_FT 166MHz fast speed @ 1.8V"
io8_166m_ft_fs_pu_1v8  "IO8_FT 166MHz fast speed @ 1.8V pullup"
io8_166m_ft_fs_pd_1v8  "IO8_FT 166MHz fast speed @ 1.8V pulldown"
io8_166m_ft_ms_1v8  "IO8_FT 166MHz med speed @ 1.8V"
io8_166m_ft_ms_pu_1v8  "IO8_FT 166MHz med speed @ 1.8V pullup"
io8_166m_ft_ms_pd_1v8  "IO8_FT 166MHz med speed @ 1.8V pulldown"
io8_166m_ft_ls_1v8  "IO8_FT 166MHz low speed @ 1.8V"
io8_166m_ft_ls_pu_1v8  "IO8_FT 166MHz low speed @ 1.8V pullup"
io8_166m_ft_ls_pd_1v8  "IO8_FT 166MHz low speed @ 1.8V pulldown"
io8_166m_ft_hs_3v3  "IO8_FT 166MHz high speed @ 3.3V"
io8_166m_ft_hs_pu_3v3  "IO8_FT 166MHz high speed @ 3.3V pullup"
io8_166m_ft_hs_pd_3v3  "IO8_FT 166MHz high speed @ 3.3V pulldown"
io8_166m_ft_fs_3v3  "IO8_FT 166MHz fast speed @ 3.3V"
io8_166m_ft_fs_pu_3v3  "IO8_FT 166MHz fast speed @ 3.3V pullup"
io8_166m_ft_fs_pd_3v3  "IO8_FT 166MHz fast speed @ 3.3V pulldown"
io8_166m_ft_ms_3v3  "IO8_FT 166MHz med speed @ 3.3V"
io8_166m_ft_ms_pu_3v3  "IO8_FT 166MHz med speed @ 3.3V pullup"
io8_166m_ft_ms_pd_3v3  "IO8_FT 166MHz med speed @ 3.3V pulldown"
io8_166m_ft_ls_3v3  "IO8_FT 166MHz low speed @ 3.3V"
io8_166m_ft_ls_pu_3v3  "IO8_FT 166MHz low speed @ 3.3V pullup"
io8_166m_ft_ls_pd_3v3  "IO8_FT 166MHz low speed @ 3.3V pulldown"
io8_166m_hslv_ft_hs_1v2  "IO8_FT 166MHz HSLV high speed @ 1.2V"
io8_166m_hslv_ft_hs_pu_1v2  "IO8_FT 166MHz HSLV high speed @ 1.2V pullup"
io8_166m_hslv_ft_hs_pd_1v2  "IO8_FT 166MHz HSLV high speed @ 1.2V pulldown"
io8_166m_hslv_ft_fs_1v2  "IO8_FT 166MHz HSLV fast speed @ 1.2V"
io8_166m_hslv_ft_fs_pu_1v2  "IO8_FT 166MHz HSLV fast speed @ 1.2V pullup"
io8_166m_hslv_ft_fs_pd_1v2  "IO8_FT 166MHz HSLV fast speed @ 1.2V pulldown"
io8_166m_hslv_ft_ms_1v2  "IO8_FT 166MHz HSLV med speed @ 1.2V"
io8_166m_hslv_ft_ms_pu_1v2  "IO8_FT 166MHz HSLV med speed @ 1.2V pullup"
io8_166m_hslv_ft_ms_pd_1v2  "IO8_FT 166MHz HSLV med speed @ 1.2V pulldown"
io8_166m_hslv_ft_ls_1v2  "IO8_FT 166MHz HSLV low speed @ 1.2V"
io8_166m_hslv_ft_ls_pu_1v2  "IO8_FT 166MHz HSLV low speed @ 1.2V pullup"
io8_166m_hslv_ft_ls_pd_1v2  "IO8_FT 166MHz HSLV low speed @ 1.2V pulldown"
io8_166m_hslv_ft_hs_1v8  "IO8_FT 166MHz HSLV high speed @ 1.8V"
io8_166m_hslv_ft_hs_pu_1v8  "IO8_FT 166MHz HSLV high speed @ 1.8V pullup"
io8_166m_hslv_ft_hs_pd_1v8  "IO8_FT 166MHz HSLV high speed @ 1.8V pulldown"
io8_166m_hslv_ft_fs_1v8  "IO8_FT 166MHz HSLV fast speed @ 1.8V"
io8_166m_hslv_ft_fs_pu_1v8  "IO8_FT 166MHz HSLV fast speed @ 1.8V pullup"
io8_166m_hslv_ft_fs_pd_1v8  "IO8_FT 166MHz HSLV fast speed @ 1.8V pulldown"
io8_166m_hslv_ft_ms_1v8  "IO8_FT 166MHz HSLV med speed @ 1.8V"
io8_166m_hslv_ft_ms_pu_1v8  "IO8_FT 166MHz HSLV med speed @ 1.8V pullup"
io8_166m_hslv_ft_ms_pd_1v8  "IO8_FT 166MHz HSLV med speed @ 1.8V pulldown"
io8_166m_hslv_ft_ls_1v8  "IO8_FT 166MHz HSLV low speed @ 1.8V"
io8_166m_hslv_ft_ls_pu_1v8  "IO8_FT 166MHz HSLV low speed @ 1.8V pullup"
io8_166m_hslv_ft_ls_pd_1v8  "IO8_FT 166MHz HSLV low speed @ 1.8V pulldown"
io8_166m_hslv_ft_hs_2v5  "IO8_FT 166MHz HSLV high speed @ 2.5V"
io8_166m_hslv_ft_hs_pu_2v5  "IO8_FT 166MHz HSLV high speed @ 2.5V pullup"
io8_166m_hslv_ft_hs_pd_2v5  "IO8_FT 166MHz HSLV high speed @ 2.5V pulldown"
io8_166m_hslv_ft_fs_2v5  "IO8_FT 166MHz HSLV fast speed @ 2.5V"
io8_166m_hslv_ft_fs_pu_2v5  "IO8_FT 166MHz HSLV fast speed @ 2.5V pullup"
io8_166m_hslv_ft_fs_pd_2v5  "IO8_FT 166MHz HSLV fast speed @ 2.5V pulldown"
io8_166m_hslv_ft_ms_2v5  "IO8_FT 166MHz HSLV med speed @ 2.5V"
io8_166m_hslv_ft_ms_pu_2v5  "IO8_FT 166MHz HSLV med speed @ 2.5V pullup"
io8_166m_hslv_ft_ms_pd_2v5  "IO8_FT 166MHz HSLV med speed @ 2.5V pulldown"
io8_166m_hslv_ft_ls_2v5  "IO8_FT 166MHz HSLV low speed @ 2.5V"
io8_166m_hslv_ft_ls_pu_2v5  "IO8_FT 166MHz HSLV low speed @ 2.5V pullup"
io8_166m_hslv_ft_ls_pd_2v5  "IO8_FT 166MHz HSLV low speed @ 2.5V pulldown"
io8_166m_i2c_ft_1v2  "IO8_FT 166MHz I2C @ 1.2V"
io8_166m_i2c_ft_pu_1v2  "IO8_FT 166MHz I2C @ 1.2V pullup"
io8_166m_i2c_ft_pd_1v2  "IO8_FT 166MHz I2C @ 1.2V pulldown"
io8_166m_i2c_ft_1v8  "IO8_FT 166MHz I2C @ 1.8V"
io8_166m_i2c_ft_pu_1v8  "IO8_FT 166MHz I2C @ 1.8V pullup"
io8_166m_i2c_ft_pd_1v8  "IO8_FT 166MHz I2C @ 1,8V pulldown"
io8_166m_i2c_ft_3v3  "IO8_FT 166MHz I2C @ 3.3V"
io8_166m_i2c_ft_pu_3v3  "IO8_FT 166MHz I2C HSLV @ 3.3V pullup"
io8_166m_i2c_ft_pd_3v3  "IO8_FT 166MHz I2C @ 3.3V pulldown"
[Model Selector] io8_100m_ft_v33
io8_ft_v33_hs_1v2  "IO8_FT_V33 high speed @ 1.2V"
io8_ft_v33_hs_pu_1v2  "IO8_FT_V33 high speed @ 1.2V pullup"
io8_ft_v33_hs_pd_1v2  "IO8_FT_V33 high speed @ 1.2V pulldown"
io8_ft_v33_fs_1v2  "IO8_FT_V33 fast speed @ 1.2V"
io8_ft_v33_fs_pu_1v2  "IO8_FT_V33 fast speed @ 1.2V pullup"
io8_ft_v33_fs_pd_1v2  "IO8_FT_V33 fast speed @ 1.2V pulldown"
io8_ft_v33_ms_1v2  "IO8_FT_V33 med speed @ 1.2V"
io8_ft_v33_ms_pu_1v2  "IO8_FT_V33 med speed @ 1.2V pullup"
io8_ft_v33_ms_pd_1v2  "IO8_FT_V33 med speed @ 1.2V pulldown"
io8_ft_v33_ls_1v2  "IO8_FT_V33 low speed @ 1.2V"
io8_ft_v33_ls_pu_1v2  "IO8_FT_V33 low speed @ 1.2V pullup"
io8_ft_v33_ls_pd_1v2  "IO8_FT_V33 low speed @ 1.2V pulldown"
io8_ft_v33_hs_1v8  "IO8_FT_V33 high speed @ 1.8V"
io8_ft_v33_hs_pu_1v8  "IO8_FT_V33 high speed @ 1.8V pullup"
io8_ft_v33_hs_pd_1v8  "IO8_FT_V33 high speed @ 1.8V pulldown"
io8_ft_v33_fs_1v8  "IO8_FT_V33 fast speed @ 1.8V"
io8_ft_v33_fs_pu_1v8  "IO8_FT_V33 fast speed @ 1.8V pullup"
io8_ft_v33_fs_pd_1v8  "IO8_FT_V33 fast speed @ 1.8V pulldown"
io8_ft_v33_ms_1v8  "IO8_FT_V33 med speed @ 1.8V"
io8_ft_v33_ms_pu_1v8  "IO8_FT_V33 med speed @ 1.8V pullup"
io8_ft_v33_ms_pd_1v8  "IO8_FT_V33 med speed @ 1.8V pulldown"
io8_ft_v33_ls_1v8  "IO8_FT_V33 low speed @ 1.8V"
io8_ft_v33_ls_pu_1v8  "IO8_FT_V33 low speed @ 1.8V pullup"
io8_ft_v33_ls_pd_1v8  "IO8_FT_V33 low speed @ 1.8V pulldown"
io8_ft_v33_hs_3v3  "IO8_FT_V33 high speed @ 3.3V"
io8_ft_v33_hs_pu_3v3  "IO8_FT_V33 high speed @ 3.3V pullup"
io8_ft_v33_hs_pd_3v3  "IO8_FT_V33 high speed @ 3.3V pulldown"
io8_ft_v33_fs_3v3  "IO8_FT_V33 fast speed @ 3.3V"
io8_ft_v33_fs_pu_3v3  "IO8_FT_V33 fast speed @ 3.3V pullup"
io8_ft_v33_fs_pd_3v3  "IO8_FT_V33 fast speed @ 3.3V pulldown"
io8_ft_v33_ms_3v3  "IO8_FT_V33 med speed @ 3.3V"
io8_ft_v33_ms_pu_3v3  "IO8_FT_V33 med speed @ 3.3V pullup"
io8_ft_v33_ms_pd_3v3  "IO8_FT_V33 med speed @ 3.3V pulldown"
io8_ft_v33_ls_3v3  "IO8_FT_V33 low speed @ 3.3V"
io8_ft_v33_ls_pu_3v3  "IO8_FT_V33 low speed @ 3.3V pullup"
io8_ft_v33_ls_pd_3v3  "IO8_FT_V33 low speed @ 3.3V pulldown"
[Define Package Model]  455-lqfp-10x10-64-ldo-230425
[Manufacturer]  Unknown
[OEM]  Unknown
[Description]  None
[Number Of Pins]  61
[Pin Numbers]
| Pin Num   Terminal Name
7 | NRST
14 | PA0
43 | PA10
44 | PA11
45 | PA12
46 | PA13
49 | PA14
50 | PA15
15 | PA1
16 | PA2
17 | PA3
20 | PA4
21 | PA5
22 | PA6
23 | PA7
41 | PA8
42 | PA9
26 | PB0
29 | PB10
33 | PB12
34 | PB13
35 | PB14
36 | PB15
27 | PB1
28 | PB2
55 | PB3
56 | PB4
57 | PB5
58 | PB6
59 | PB7
61 | PB8
62 | PB9
8 | PC0
51 | PC10
52 | PC11
53 | PC12
2 | PC13
3 | PC14-OSC32_IN
4 | PC15-OSC32_OUT
9 | PC1
10 | PC2
11 | PC3
24 | PC4
25 | PC5
37 | PC6
38 | PC7
39 | PC8
40 | PC9
54 | PD2
5 | PH0-OSC_IN
6 | PH1-OSC_OUT
60 | PH3-BOOT0
30 | VCAP
1 | VBAT
32 | VDD
64 | VDD
19 | VDD
48 | VDDUSB
13 | VDDA
18 | VSS
12 | VSSA
|[Merged Pins]  18
|31  |  VSS
|47  |  VSS
|63  |  VSS
[Model Data]
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[End Model Data]
[End Package Model]
| Models and submodels in the file (208): io8_100m_ft_hs_1v2 (I/O), io8_100m_ft_hs_pu_1v2 (I/O), io8_100m_ft_hs_pd_1v2 (I/O), io8_100m_ft_fs_1v2 (I/O), io8_100m_ft_fs_pu_1v2 (I/O), io8_100m_ft_fs_pd_1v2 (I/O), io8_100m_ft_ms_1v2 (I/O), io8_100m_ft_ms_pu_1v2 (I/O), io8_100m_ft_ms_pd_1v2 (I/O), io8_100m_ft_ls_1v2 (I/O), io8_100m_ft_ls_pu_1v2 (I/O), io8_100m_ft_ls_pd_1v2 (I/O), io8_100m_ft_hs_1v8 (I/O), io8_100m_ft_hs_pu_1v8 (I/O), io8_100m_ft_hs_pd_1v8 (I/O), io8_100m_ft_fs_1v8 (I/O), io8_100m_ft_fs_pu_1v8 (I/O), io8_100m_ft_fs_pd_1v8 (I/O), io8_100m_ft_ms_1v8 (I/O), io8_100m_ft_ms_pu_1v8 (I/O), io8_100m_ft_ms_pd_1v8 (I/O), io8_100m_ft_ls_1v8 (I/O), io8_100m_ft_ls_pu_1v8 (I/O), io8_100m_ft_ls_pd_1v8 (I/O), io8_100m_ft_hs_3v3 (I/O), io8_100m_ft_hs_pu_3v3 (I/O), io8_100m_ft_hs_pd_3v3 (I/O), io8_100m_ft_fs_3v3 (I/O), io8_100m_ft_fs_pu_3v3 (I/O), io8_100m_ft_fs_pd_3v3 (I/O), io8_100m_ft_ms_3v3 (I/O), io8_100m_ft_ms_pu_3v3 (I/O), io8_100m_ft_ms_pd_3v3 (I/O), io8_100m_ft_ls_3v3 (I/O), io8_100m_ft_ls_pu_3v3 (I/O), io8_100m_ft_ls_pd_3v3 (I/O), io8_100m_hslv_ft_hs_1v2 (I/O), io8_100m_hslv_ft_hs_pu_1v2 (I/O), io8_100m_hslv_ft_hs_pd_1v2 (I/O), io8_100m_hslv_ft_fs_1v2 (I/O), io8_100m_hslv_ft_fs_pu_1v2 (I/O), io8_100m_hslv_ft_fs_pd_1v2 (I/O), io8_100m_hslv_ft_ms_1v2 (I/O), io8_100m_hslv_ft_ms_pu_1v2 (I/O), io8_100m_hslv_ft_ms_pd_1v2 (I/O), io8_100m_hslv_ft_ls_1v2 (I/O), io8_100m_hslv_ft_ls_pu_1v2 (I/O), io8_100m_hslv_ft_ls_pd_1v2 (I/O), io8_100m_hslv_ft_hs_1v8 (I/O), io8_100m_hslv_ft_hs_pu_1v8 (I/O), io8_100m_hslv_ft_hs_pd_1v8 (I/O), io8_100m_hslv_ft_fs_1v8 (I/O), io8_100m_hslv_ft_fs_pu_1v8 (I/O), io8_100m_hslv_ft_fs_pd_1v8 (I/O), io8_100m_hslv_ft_ms_1v8 (I/O), io8_100m_hslv_ft_ms_pu_1v8 (I/O), io8_100m_hslv_ft_ms_pd_1v8 (I/O), io8_100m_hslv_ft_ls_1v8 (I/O), io8_100m_hslv_ft_ls_pu_1v8 (I/O), io8_100m_hslv_ft_ls_pd_1v8 (I/O), io8_100m_hslv_ft_hs_2v5 (I/O), io8_100m_hslv_ft_hs_pu_2v5 (I/O), io8_100m_hslv_ft_hs_pd_2v5 (I/O), io8_100m_hslv_ft_fs_2v5 (I/O), io8_100m_hslv_ft_fs_pu_2v5 (I/O), io8_100m_hslv_ft_fs_pd_2v5 (I/O), io8_100m_hslv_ft_ms_2v5 (I/O), io8_100m_hslv_ft_ms_pu_2v5 (I/O), io8_100m_hslv_ft_ms_pd_2v5 (I/O), io8_100m_hslv_ft_ls_2v5 (I/O), io8_100m_hslv_ft_ls_pu_2v5 (I/O), io8_100m_hslv_ft_ls_pd_2v5 (I/O), io8_166m_ft_hs_1v2 (I/O), io8_166m_ft_hs_pu_1v2 (I/O), io8_166m_ft_hs_pd_1v2 (I/O), io8_166m_ft_fs_1v2 (I/O), io8_166m_ft_fs_pu_1v2 (I/O), io8_166m_ft_fs_pd_1v2 (I/O), io8_166m_ft_ms_1v2 (I/O), io8_166m_ft_ms_pu_1v2 (I/O)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
